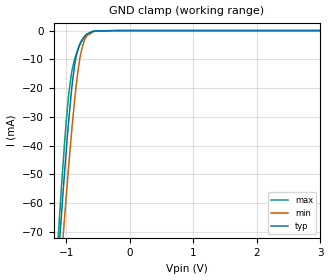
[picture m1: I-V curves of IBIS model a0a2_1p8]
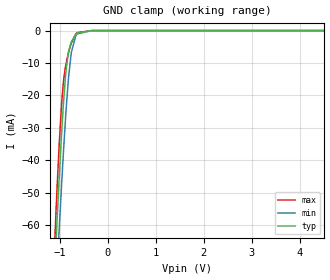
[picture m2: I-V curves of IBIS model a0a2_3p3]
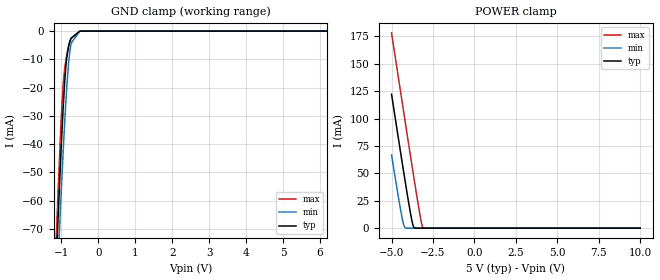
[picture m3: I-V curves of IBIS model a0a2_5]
|Texas Instruments Incorporated
| TCA9535 Low-Voltage 16-Bit I2C and SMBus Low-Power I/O
| Expander with Interrupt Output and Configuration Registers
| Marketing part#   Digital Voltage Range   Package-type   #pins
| TCA9535DBR   1.65V-5.5V   SSOP   24
| TCA9535DBT   1.65V-5.5V   SSOP   24
| TCA9535PWR   1.65V-5.5V   TSSOP   24
| TCA9535RGER   1.65V-5.5V   VQFN   24
| TCA9535RTWR   1.65V-5.5V   WQFN   24
[IBIS Ver]   4.1
[File name]   tca9535.ibs
[File Rev]   1.0
[Date]   11/16/2016
[Source]
| Texas Instruments Incorporated.
| Analog-eLab Design Center, HPA
| 12500 TI Blvd
| Dallas, TX -75243
[Notes]   Revision History:
| Rev 1.0: 11/16/2016
| - Relative Part of TCA9555
| - Initial version of the model
| - Model generated from simulations in SPECTRE
| - Model matched to SPICE simulation
| - C_comp although listed in numerical order of value are
|   obtained from varying PVT conditions. For PVT conditions for
|   each specific value refer the buffer description under
|   respective [Model]. IBIS model user is responsible for using
|   appropriate C_comp to simulate for Signal Integrity.
|* EXCEPTION:   *
|* - For models io_*,there will be leakage in ground clamp IV table   *
|*   because of resistor Rpullup connected to pad.   *
|* - For model io_*,pullup and pulldown IV tables does not pass through 0   *
|*   because of transistors(MN1-MN8) and resistor Rpullup connected to pad. *
|* - For model intz_*,pulldown IV tables does not pass through 0   *
|*   because of pulldown transistors(MN1-MN3 and MN11) connected to pad.   *
|* - For model sda_*,pulldown IV tables does not pass through 0   *
|*   because of pulldown transistors(MN1-MN4) connected to pad.   *
[Disclaimer]
| This model is designed as an aid for customers of Texas Instruments.
| TI and its licensors and suppliers make no warranties, either expressed
| or implied, with respect to this  model, including the warranties of
| merchantability or fitness for a particular purpose. The model is
| provided solely on an "as is" basis. The entire risk as to its quality
| and performance is with the customer.
[Copyright]
(C) Copyright 2016 Texas Instruments Incorporated.All rights reserved.
|   TCA9535DB
[Component]   TCA9535DB
[Manufacturer]   TI
[Package]   |24 SSOP  -  DB  package
|   typ   min   max
R_pkg   0.1   0.08   0.12
L_pkg   1.0nH   0.8nH   1.2nH
C_pkg   0.2pF   0.16pF   0.24pF
[Pin]  signal_name   model_name   R_pin   L_pin   C_pin
1   _INT   intz   NA   NA   NA
2   A1   a1   NA   NA   NA
3   A2   a0a2   NA   NA   NA
4   P00   io   NA   NA   NA
5   P01   io   NA   NA   NA
6   P02   io   NA   NA   NA
7   P03   io   NA   NA   NA
8   P04   io   NA   NA   NA
9   P05   io   NA   NA   NA
10   P06   io   NA   NA   NA
11   P07   io   NA   NA   NA
12   GND   gnd   NA   NA   NA
13   P10   io   NA   NA   NA
14   P11   io   NA   NA   NA
15   P12   io   NA   NA   NA
16   P13   io   NA   NA   NA
17   P14   io   NA   NA   NA
18   P15   io   NA   NA   NA
19   P16   io   NA   NA   NA
20   P17   io   NA   NA   NA
21   A0   a0a2   NA   NA   NA
22   SCL   scl   NA   NA   NA
23   SDA   sda   NA   NA   NA
24   VCC   power   NA   NA   NA
|   TCA9535PW
[Component]   TCA9535PW
[Manufacturer]   TI
[Package]   |24 TSSOP  -  PW  package
|   typ   min   max
R_pkg   0.1   0.08   0.12
L_pkg   1.0nH   0.8nH   1.2nH
C_pkg   0.2pF   0.16pF   0.24pF
[Pin]  signal_name   model_name   R_pin   L_pin   C_pin
1   _INT   intz   NA   NA   NA
2   A1   a1   NA   NA   NA
3   A2   a0a2   NA   NA   NA
4   P00   io   NA   NA   NA
5   P01   io   NA   NA   NA
6   P02   io   NA   NA   NA
7   P03   io   NA   NA   NA
8   P04   io   NA   NA   NA
9   P05   io   NA   NA   NA
10   P06   io   NA   NA   NA
11   P07   io   NA   NA   NA
12   GND   gnd   NA   NA   NA
13   P10   io   NA   NA   NA
14   P11   io   NA   NA   NA
15   P12   io   NA   NA   NA
16   P13   io   NA   NA   NA
17   P14   io   NA   NA   NA
18   P15   io   NA   NA   NA
19   P16   io   NA   NA   NA
20   P17   io   NA   NA   NA
21   A0   a0a2   NA   NA   NA
22   SCL   scl   NA   NA   NA
23   SDA   sda   NA   NA   NA
24   VCC   power   NA   NA   NA
|   TCA9535RTW
[Component]   TCA9535RTW
[Manufacturer]   TI
[Package]   |24 WQFN  -  RTW  package
|   typ   min   max
R_pkg   0.1   0.08   0.12
L_pkg   1.0nH   0.8nH   1.2nH
C_pkg   0.2pF   0.16pF   0.24pF
[Pin]  signal_name   model_name   R_pin   L_pin   C_pin
1   P00   io   NA   NA   NA
2   P01   io   NA   NA   NA
3   P02   io   NA   NA   NA
4   P03   io   NA   NA   NA
5   P04   io   NA   NA   NA
6   P05   io   NA   NA   NA
7   P06   io   NA   NA   NA
8   P07   io   NA   NA   NA
9   GND   gnd   NA   NA   NA
10   P10   io   NA   NA   NA
11   P11   io   NA   NA   NA
12   P12   io   NA   NA   NA
13   P13   io   NA   NA   NA
14   P14   io   NA   NA   NA
15   P15   io   NA   NA   NA
16   P16   io   NA   NA   NA
17   P17   io   NA   NA   NA
18   A0   a0a2   NA   NA   NA
19   SCL   scl   NA   NA   NA
20   SDA   sda   NA   NA   NA
21   VCC   power   NA   NA   NA
22   _INT   intz   NA   NA   NA
23   A1   a1   NA   NA   NA
24   A2   a0a2   NA   NA   NA
|   TCA9535RGE
[Component]   TCA9535RGE
[Manufacturer]   TI
[Package]   |24 VQFN  -  RGE  package
|   typ   min   max
R_pkg   0.1   0.08   0.12
L_pkg   1.0nH   0.8nH   1.2nH
C_pkg   0.2pF   0.16pF   0.24pF
[Pin]  signal_name   model_name   R_pin   L_pin   C_pin
1   P00   io   NA   NA   NA
2   P01   io   NA   NA   NA
3   P02   io   NA   NA   NA
4   P03   io   NA   NA   NA
5   P04   io   NA   NA   NA
6   P05   io   NA   NA   NA
7   P06   io   NA   NA   NA
8   P07   io   NA   NA   NA
9   GND   gnd   NA   NA   NA
10   P10   io   NA   NA   NA
11   P11   io   NA   NA   NA
12   P12   io   NA   NA   NA
13   P13   io   NA   NA   NA
14   P14   io   NA   NA   NA
15   P15   io   NA   NA   NA
16   P16   io   NA   NA   NA
17   P17   io   NA   NA   NA
18   A0   a0a2   NA   NA   NA
19   SCL   scl   NA   NA   NA
20   SDA   sda   NA   NA   NA
21   VCC   power   NA   NA   NA
22   _INT   intz   NA   NA   NA
23   A1   a1   NA   NA   NA
24   A2   a0a2   NA   NA   NA
|   Model Selectors
[Model Selector] a0a2
a0a2_1p8   1.8V  digital Input
a0a2_3p3   3.3V  digital Input
a0a2_5   5.0V  digital Input
[Model Selector] a1
a1_1p8   1.8V  digital Input
a1_3p3   3.3V  digital Input
a1_5   5.0V  digital Input
[Model Selector] scl
scl_1p8   1.8V  digital Input
scl_3p3   3.3V  digital Input
scl_5   5.0V  digital Input
[Model Selector] io
io_1p8   1.8V  digital I/O
io_3p3   3.3V  digital I/O
io_5   5.0V  digital I/O
[Model Selector] intz
intz_1p8   1.8V  digital Open_sink
intz_3p3   3.3V  digital Open_sink
intz_5   5.0V  digital Open_sink
[Model Selector] sda
sda_1p8   1.8V  digital I/O_open_drain
sda_3p3   3.3V  digital I/O_open_drain
sda_5   5.0V  digital I/O_open_drain
| Models and submodels in the file (18): a0a2_1p8 (Input), a0a2_3p3 (Input), a0a2_5 (Input), a1_1p8 (Input), a1_3p3 (Input), a1_5 (Input), scl_1p8 (Input), scl_3p3 (Input), scl_5 (Input), io_1p8 (I/O), io_3p3 (I/O), io_5 (I/O), intz_1p8 (Open_sink), intz_3p3 (Open_sink), intz_5 (Open_sink), sda_1p8 (I/O_open_drain), sda_3p3 (I/O_open_drain), sda_5 (I/O_open_drain)
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|   a0a2_1p8 Model
[Model]   a0a2_1p8
Model_type   Input
Vinl = 0.54
Vinh = 1.26
|   typ   min   max
|   (nom PVT)   (fast PVT)   (slow PVT)
C_comp   1.340e-12   1.280e-12   1.472e-12
[Model spec]
|subparameter
Vinl   0.54   0.495   0.585
Vinh   1.26   1.155   1.365
| Where nom  PVT is Nominal Process, 1.8V, 27C
|   Fast PVT is Strong Process,  1.95V, -40C
|   Slow PVT is Weak Process,   1.65V, 100C
[Voltage Range]   1.8   1.65   1.95
|Junction Temperature
[Temperature Range]   27   100   -40
[Power Clamp Reference]   1.8   1.65   1.95
[GND Clamp Reference]   0   0   0
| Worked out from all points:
|   GND clamp passes 1 mA (typ) near -0.65 V on its own axis
[GND Clamp]
|   Voltage   I(typ)   I(min)   I(max)
-1.8V     -319.1mA   -317.4mA   -335mA
-1.121V   -78.48mA   -93.12mA   -70.07mA
-1.071V   -62.62mA   -77.98mA   -53.03mA
-1.031V   -50.81mA   -66.56mA   -40.68mA
-961.2mV  -31.35mA   -47.09mA   -22.26mA
-918.6mV  -21.23mA   -36.09mA   -15.04mA
-871.8mV  -12.58mA   -25.07mA   -10.36mA
-824.4mV  -7.103mA   -15.61mA   -7.146mA
-763.8mV  -3.621mA   -7.099mA   -4.039mA
-675mV    -1.238mA   -1.806mA   -1.236mA
-180mV    0A         -74.39nA   0A
3.6V      0A         0A         0A
[POWER Clamp]
|   Voltage   I(typ)   I(min)   I(max)
-1.8V     0A         0A         0A
0V        0A         0A         0A
3.6V      0A         0A         0A
|   a0a2_3p3 Model
[Model]   a0a2_3p3
Model_type   Input
Vinl = 0.99
Vinh = 2.31
|   typ   min   max
|   (nom PVT)   (fast PVT)   (slow PVT)
C_comp   1.371e-12   1.310e-12   1.508e-12
[Model spec]
|subparameter
Vinl   0.99   0.90   1.08
Vinh   2.31   2.10   2.52
| Where nom  PVT is Nominal Process, 3.3V, 27C
|   Fast PVT is Strong Process,  3.6V, -40C
|   Slow PVT is Weak Process,   3V, 100C
[Voltage Range]   3.3   3   3.6
|Junction Temperature
[Temperature Range]   27   100   -40
[Power Clamp Reference]   3.3   3   3.6
[GND Clamp Reference]   0   0   0
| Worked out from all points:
|   GND clamp passes 1 mA (typ) near -0.66 V on its own axis
[GND Clamp]
|   Voltage   I(typ)   I(min)   I(max)
-3.3V     -909.2mA   -865.8mA   -978.8mA
-1.219V   -110mA     -122.9mA   -104.4mA
-1.082V   -65.76mA   -81.04mA   -56.33mA
-1.071V   -62.25mA   -77.67mA   -52.6mA
-1.014V   -45.33mA   -61.23mA   -35.1mA
-963.6mV  -31.58mA   -47.37mA   -22.42mA
-927.3mV  -22.81mA   -37.93mA   -16mA
-864.6mV  -11.33mA   -23.22mA   -9.689mA
-819mV    -6.554mA   -14.45mA   -6.733mA
-762mV    -3.494mA   -6.78mA    -3.892mA
-639mV    -707.5uA   -1.021mA   -634.7uA
6.6V      0A         0A         0A
[POWER Clamp]
|   Voltage   I(typ)   I(min)   I(max)
-3.3V     0A         0A         0A
0V        0A         0A         0A
6.6V      0A         0A         0A
|   a0a2_5 Model
[Model]   a0a2_5
Model_type   Input
Vinl = 1.5
Vinh = 3.5
|   typ   min   max
|   (nom PVT)   (fast PVT)   (slow PVT)
C_comp   1.404e-12   1.340e-12   1.546e-12
[Model spec]
|subparameter
Vinl   1.5   1.35   1.65
Vinh   3.5   3.15   3.85
| Where nom  PVT is Nominal Process, 5V, 27C
|   Fast PVT is Strong Process,  5.5V, -40C
|   Slow PVT is Weak Process,   4.5V, 100C
[Voltage Range]   5   4.5   5.5
|Junction Temperature
[Temperature Range]   27   100   -40
[Power Clamp Reference]   5   4.5   5.5
[GND Clamp Reference]   0   0   0
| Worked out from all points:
|   GND clamp passes 1 mA (typ) near -0.59 V on its own axis
|   POWER clamp passes 1 mA (typ) near -3.66 V on its own axis
[GND Clamp]
|   Voltage   I(typ)   I(min)   I(max)
-5V       -1.602A    -1.516A    -1.726A
-1.128V   -79.57mA   -94.26mA   -71.13mA
-1.103V   -71.65mA   -86.73mA   -62.58mA
-1.089V   -67.43mA   -82.7mA    -58.05mA
-1.007V   -42.86mA   -58.84mA   -32.61mA
-946.5mV  -26.89mA   -42.47mA   -18.74mA
-902.5mV  -17.3mA    -31.47mA   -12.77mA
-845mV    -8.747mA   -18.91mA   -8.208mA
-801.5mV  -5.272mA   -11.45mA   -5.669mA
-734mV    -2.51mA    -4.333mA   -2.746mA
-500mV    -48.27uA   -92.87uA   -25.42uA
10V       0A         0A         0A
[POWER Clamp]
|   Voltage   I(typ)   I(min)   I(max)
-5V       122.2mA    66.83mA    178.2mA
-4.519V   75.31mA    22.22mA    130.6mA
-4.343V   58.41mA    7.966mA    113.4mA
-4.235V   48.11mA    1.854mA    102.8mA
-4.15V    40.09mA    219.4uA    94.43mA
-3.865V   14.26mA    45.34nA    66.64mA
-3.71V    2.889mA    11.14nA    51.65mA
-3.61V    172.9uA    10.17nA    42.06mA
-3.272V   0A         0A         10.96mA
-3.163V   0A         0A         2.802mA
-3.091V   0A         0A         279.9uA
10V       0A         0A         0A
